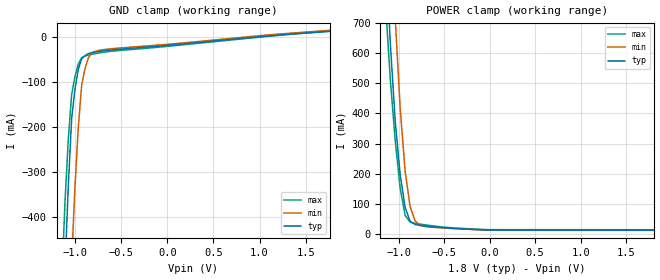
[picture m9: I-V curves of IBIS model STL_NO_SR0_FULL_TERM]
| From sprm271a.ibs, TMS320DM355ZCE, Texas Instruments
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|   Model Cell STL_NO_SR0_FULL_TERM
[Model]   STL_NO_SR0_FULL_TERM
Model_type   Input
Polarity   Non-Inverting
Vinl =  0.80
Vinh =  1.00
C_comp   2.680301p   2.549919p   2.900942p
[Model Spec]
Vinl   0.80   0.71   0.89
Vinh   1.00   0.91   1.09
[Temperature Range]   25   125   -40
[Voltage Range]   1.8   1.62   1.89
[POWER_clamp]
|   voltage   I(typ)   I(min)   I(max)
-1.8V     6.875A     7.433A     6.581A
-1.127V   866.7mA    1.361A     691.3mA
-1.109V   751.5mA    1.223A     603.3mA
-1.091V   636.4mA    1.086A     515.3mA
-1.036V   375.7mA    718mA      311.6mA
-1.018V   316.4mA    618mA      258.6mA
-981.8mV  198mA      417.9mA    152.7mA
-927.3mV  88.88mA    208.3mA    62.61mA
-872.7mV  43.6mA     92.19mA    40.63mA
-818.2mV  32.75mA    44.78mA    36.42mA
-654.5mV  26.28mA    24.22mA    29.56mA
1.8V      14.02mA    13.57mA    15.44mA
[GND_clamp]
|   voltage   I(typ)   I(min)   I(max)
-1.8V     -6.676A    -7.172A    -6.433A
-1.145V   -752mA     -1.249A    -557.1mA
-1.109V   -522.5mA   -980.7mA   -370.6mA
-1.073V   -332.3mA   -731.7mA   -227.5mA
-1.036V   -181.6mA   -501.6mA   -128mA
-1V       -115.5mA   -331.5mA   -86.97mA
-963.6mV  -70.82mA   -199.5mA   -59.32mA
-927.3mV  -47.6mA    -105.5mA   -45.05mA
-890.9mV  -40.63mA   -69.27mA   -41.79mA
-854.5mV  -36.07mA   -45.68mA   -39.37mA
-745.5mV  -31.6mA    -29.15mA   -35.11mA
1.764V    13.51mA    15.68mA    13.56mA
